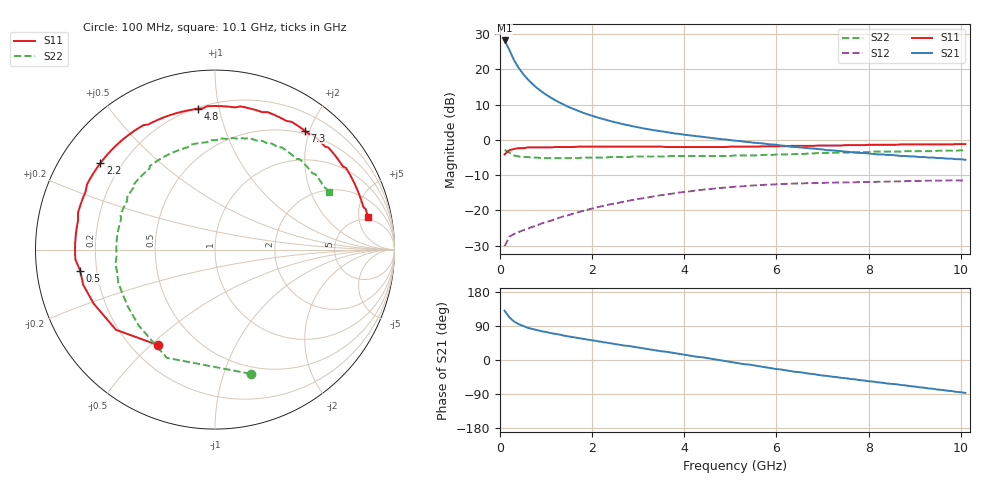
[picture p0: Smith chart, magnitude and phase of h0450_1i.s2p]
!HBFP-0450
!S and NOISE PARAMETERS at Vce=1V  Ic=70mA.  LAST UPDATED  09-04-98
# GHZ S MA R  50
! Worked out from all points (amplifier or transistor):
!   101 points, 100 MHz to 10.1 GHz, reference 50 ohm
!   highest |S21| = 28.2 dB at 100 MHz (marker M1)
!   |S21| within 3 dB of that: start of sweep to 214.2 MHz
!   unconditionally stable (mu >= 1): 1.887 GHz to end of sweep
!   at 1.7 GHz: K = 0.97, MSG = 14.4 dB, |S12| = -20.5 dB
!   at 5.1 GHz: K = 1.09, MAG = 4.7 dB, |S12| = -13.3 dB
!   at 10.1 GHz: K = 1.09, MAG = 1.1 dB, |S12| = -11.5 dB
!   lowest NFmin = 1.96 dB at 1.8 GHz
!   S11 on the Smith chart (normalised r, x): 100 MHz: 0.30, -0.53; 500 MHz: 0.14, -0.08; 2.2 GHz: 0.12, +0.33; 4.8 GHz: 0.21, +0.86; 7.3 GHz: 0.45, +1.92; 10.1 GHz: 4.43, +6.59
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0.1  0.62 -121.0  25.65 130.0  0.031 49.0  0.72 -74.0
0.2  0.71 -141.0  19.03 113.0  0.042 37.0  0.66 -114.0
0.3  0.74 -156.0  13.67 102.0  0.046 32.0  0.6 -135.0
0.4  0.76 -165.0  10.58 95.0  0.049 32.0  0.58 -147.0
0.5  0.76 -171.0  8.61 90.0  0.052 32.0  0.57 -156.0
0.6  0.78 -176.0  7.25 85.0  0.055 32.0  0.57 -161.0
0.7  0.78 -180.0  6.22 82.0  0.058 33.0  0.56 -167.0
0.8  0.78 177.0  5.46 79.0  0.061 34.0  0.56 -172.0
0.9  0.78 173.0  4.85 76.0  0.065 35.0  0.55 -176.0
1.1  0.78 168.0  3.97 71.0  0.071 36.0  0.55 177.0
1.3  0.79 163.0  3.36 67.0  0.079 37.0  0.55 172.0
1.5  0.79 158.0  2.9 62.0  0.086 37.0  0.55 167.0
1.8  0.8 151.0  2.42 56.0  0.098 36.0  0.56 160.0
2.2  0.8 143.0  2 48.0  0.114 33.0  0.56 153.0
2.7  0.8 134.0  1.65 38.0  0.133 29.0  0.57 144.0
3.5  0.8 120.0  1.32 23.0  0.164 20.0  0.58 131.0
4.8  0.79 97.0  1.02 -1.0  0.208 2.0  0.59 109.0
5.1  0.8 91.0  0.97 -7.0  0.216 -3.0  0.6 103.0
6.8  0.82 61.0  0.75 -37.0  0.243 -28.0  0.64 75.0
7.3  0.83 53.0  0.7 -45.0  0.248 -35.0  0.66 67.0
8.5  0.85 35.0  0.61 -63.0  0.256 -51.0  0.68 51.0
10.1  0.87 12.0  0.52 -87.0  0.265 -74.0  0.71 27.0
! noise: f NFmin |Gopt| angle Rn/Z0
1.8  1.96  0.69  -150  0.12
2  1.99  0.69  -147  0.13
2.5  2.1  0.68  -137  0.23
3.5  2.39  0.7  -120  0.46
4  2.57  0.71  -110  0.67
5  2.77  0.73  -91  1.12
5.5  2.96  0.75  -82  1.49
7  3.29  0.78  -55  2.76
8  3.57  0.8  -40  3.7
10  4.03  0.8  -11  5.28
